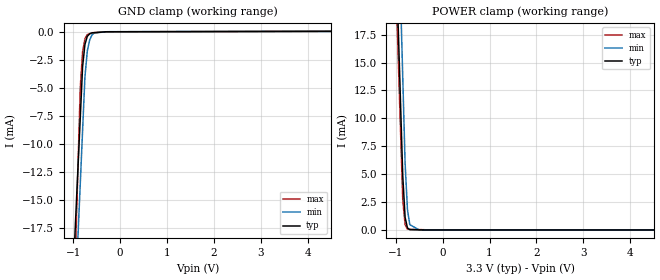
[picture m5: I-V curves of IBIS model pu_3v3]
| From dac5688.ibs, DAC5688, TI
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[Model] pu_3v3
Model_type Input
Vinl = 1.00000V
Vinh = 2.30000V
C_comp 620.000fF 620.000fF 620.000fF
| variable typ   min   max
[Voltage Range] 3.30000V 3.00000V 3.60000V
[POWER Clamp Reference] 3.30000V 3.00000V 3.60000V
[GND Clamp Reference] 0.00000V 0.00000V 0.00000V
[Temperature Range]   25   85   -40
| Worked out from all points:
|   GND clamp passes 1 mA (typ) near -0.74 V on its own axis
|   POWER clamp passes 1 mA (typ) near -0.79 V on its own axis
[GND Clamp]
-3.3V     -232.5mA   -247.9mA   -362.5mA
-850mV    -7.707mA   -13.6mA    -5.005mA
-800mV    -3.12mA    -8.819mA   -1.818mA
-750mV    -1.149mA   -4.037mA   -627.3uA
-700mV    -427.6uA   -1.738mA   -265.9uA
-650mV    -207uA     -766uA     -186uA
-600mV    -118.1uA   -302.5uA   -106.1uA
-550mV    -101.9uA   -131uA     -92.81uA
-300mV    -21.16uA   -26.68uA   -26.58uA
-275mV    -20.95uA   -16.25uA   -26.34uA
6.6V      35.71uA    30.8uA     41.13uA
[POWER Clamp]
-3.3V     342.4mA    390.7mA    324.8mA
-1.05V    32.4mA     44.48mA    28.98mA
-850mV    4.854mA    13.7mA     2.683mA
-800mV    1.133mA    6.01mA     477.3uA
-750mV    184.6uA    1.845mA    69.26uA
-700mV    26.17uA    475.3uA    62.66uA
-500mV    11.21uA    6.121uA    36.28uA
6.6V      0A         0A         0A
